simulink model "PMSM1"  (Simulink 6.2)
settings: Solver=ode45  StartTime=0  StopTime=0.2  FixedStep=0.000001  RelTol=1e-3
undefined symbols (not defined in the file or in its folder): di, DiscIntNeverNeededParam, Element, J, Lsx, Lsy, p, Psim, Rs, Symmetrized, Ts, Udc, Warning
libraries: simulink x4

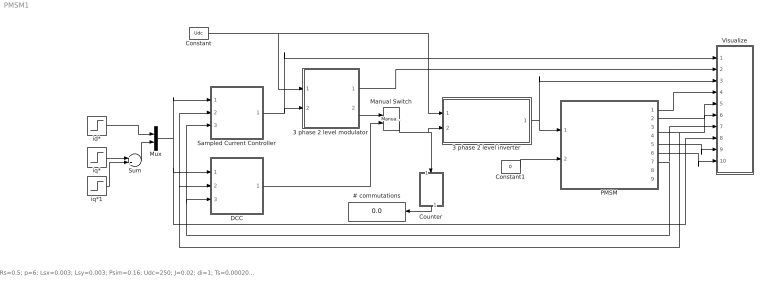
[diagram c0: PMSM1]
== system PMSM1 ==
  note: Rs=0.5; p=6; Lsx=0.003; Lsy=0.003; Psim=0.16; Udc=250; J=0.02; di=1; Ts=0.0002083;
  # commutations : Display
  3 phase 2 level inverter : Subsystem
  3 phase 2 level modulator : Subsystem  mask{type=Symmetrized, Random=Fixed frequency, Ts=Ts}
      mask prompts: type "Sinus, Symmetrized or Minimum switch modulation"; Random "Fixed or random modulation?"; Ts "Sampling interval"
      mask help: Carrier Wave modulator that uses either fixed frequency modulation or random modulation. The fixed frequency modulation uses 1/(2Ts) as modulation frequency. The random modulation selects the modulatio frequency by random every sampling instant. The selection uses either 1/Ts, 1/(2Ts) or 1/(3Ts) as carrier wave frequency.
  Constant : Constant  Value=Udc
  Constant1 : Constant  Value=0
  Counter : Subsystem  Orientation=down
  DCC : Subsystem
  Manual Switch : simulink/Signal Routing/Manual Switch  sw=1  action=0
  Mux : Mux  Inputs=2
  PMSM : Subsystem  mask{Psim=Psim, p=p, Rs=Rs, isy=[0 1], psisy=[0 Lsy], isx=[0 1], psisx=[0 Lsx], J=J}
      mask prompts: p "Number of poles"; Rs "Stator resistance"; isy "y-axis current vector"; psisy "y-axis flux vector"; isx "x-axis current vector"; psisx "x-axis flux vector"; J "Inertia"
  Sampled Current Controller : Subsystem  mask{R=Rs, Lx=Lsx, Ly=Lsy, Kp=[(Lsx/Ts+Rs/2) (Lsy/Ts+Rs/2)]', Ti=[(Lsx/Rs+Ts/2) (Lsy/Rs+Ts/2)]', Ts=Ts, Umax=Udc, Umin=-Udc, SlowFast=Fast computer}
      mask prompts: R "Load resistance"; Lx "x-axis load inductance"; Ly "y-axis load inductance"; Kp "Controller gain"; Ti "Integral Time Constant"; Ts "Sampling time [s]"; Umax "Max output signal"; Umin "Min output signal"; SlowFast "Controller type"
  Sum : Sum
  Visualize : Subsystem
  id* : Step  Time=0.0105  After=0  SampleTime=0
  iq* : Step  Time=0.0055  After=10  SampleTime=0
  iq*1 : Step  Time=0.05  After=-5  SampleTime=0
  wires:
  3 phase 2 level inverter/1(va,b,c) -> Visualize/3(v), PMSM/1(vabc)
  Sampled Current Controller/1(u*) -> 3 phase 2 level modulator/2(uabc*), Visualize/1(u*)
  Constant/1 -> 3 phase 2 level inverter/1(Udc), 3 phase 2 level modulator/1(Udc)
  Counter/1(#) -> # commutations/1
  3 phase 2 level modulator/2(sa,b,c) -> Manual Switch/1
  Manual Switch/1 -> 3 phase 2 level inverter/2(sa,b,c), Counter/1(sa,b,c)
  DCC/1(sa,b,c) -> Manual Switch/2
  3 phase 2 level modulator/1(mod) -> Visualize/2(mod)
  id*/1 -> Mux/1
  Mux/1 -> Sampled Current Controller/1(Ref_dq), DCC/1(Ref_dq), Visualize/8(i*dq)
  PMSM/7(theta_el) -> Visualize/7(theta), Sampled Current Controller/3(thetaR), DCC/3(thetaR)
  Constant1/1 -> PMSM/2(Tl)
  PMSM/1(uabc) -> Visualize/4("u ")
  PMSM/4(is) -> Visualize/6(i), DCC/2(Act_ab), Sampled Current Controller/2(Act_ab)
  PMSM/2(exy) -> Visualize/5(e)
  PMSM/5(T_mech) -> Visualize/9(Tmech)
  PMSM/6(w_mech) -> Visualize/10(wmech)
  iq*/1 -> Sum/1
  iq*1/1 -> Sum/2
  Sum/1 -> Mux/2

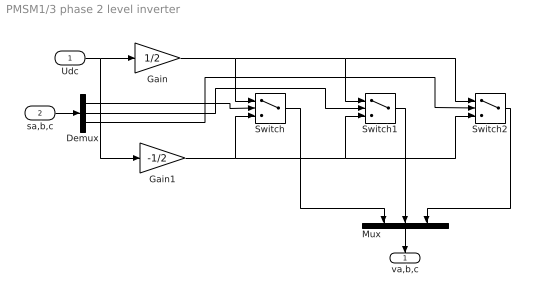
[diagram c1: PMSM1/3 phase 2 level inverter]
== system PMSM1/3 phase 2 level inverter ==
  Udc : Inport  Port=1  LatchInput=off
  sa,b,c : Inport  Port=2  LatchInput=off
  Demux : Demux  Outputs=3
  Gain : Gain  Gain=1/2
  Gain1 : Gain  Gain=-1/2
  Mux : Mux  Orientation=down  Inputs=3
  Switch : Switch
  Switch1 : Switch
  Switch2 : Switch
  va,b,c : Outport  Orientation=down  InitialOutput=0
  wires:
  Gain/1 -> Switch/1, Switch1/1, Switch2/1
  Gain1/1 -> Switch/3, Switch1/3, Switch2/3
  Udc/1 -> Gain1/1, Gain/1
  sa,b,c/1 -> Demux/1
  Demux/1 -> Switch/2
  Demux/2 -> Switch1/2
  Demux/3 -> Switch2/2
  Switch/1 -> Mux/1
  Switch1/1 -> Mux/2
  Switch2/1 -> Mux/3
  Mux/1 -> va,b,c/1

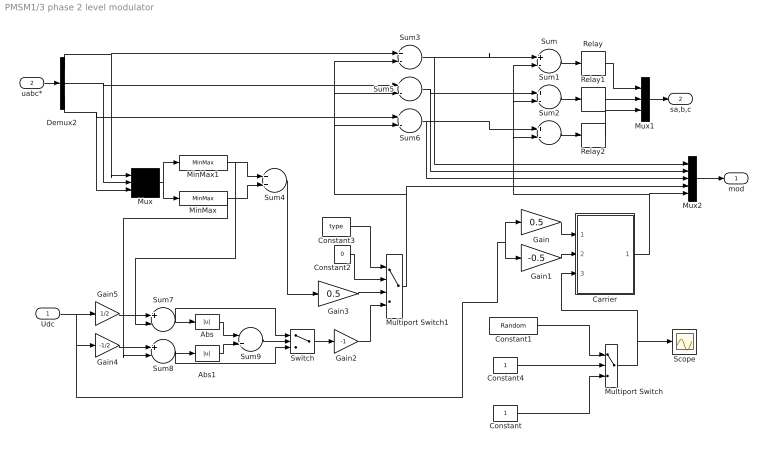
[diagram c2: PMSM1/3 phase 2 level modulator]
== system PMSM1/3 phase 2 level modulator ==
  Udc : Inport  Port=1  LatchInput=off
  uabc* : Inport  Port=2  LatchInput=off
  Abs : Abs
  Abs1 : Abs
  Carrier : Subsystem
  Constant : Constant
  Constant1 : Constant  Value=Random
  Constant2 : Constant  Value=0
  Constant3 : Constant  Value=type
  Constant4 : Constant
  Demux2 : Demux  Outputs=3
  Gain : Gain  Gain=0.5
  Gain1 : Gain  Gain=-0.5
  Gain2 : Gain  Gain=-1
  Gain3 : Gain  Gain=0.5
  Gain4 : Gain  Gain=-1/2
  Gain5 : Gain  Gain=1/2
  MinMax : MinMax
  MinMax1 : MinMax  Function=max
  Multiport Switch : MultiPortSwitch  Inputs=2
  Multiport Switch1 : MultiPortSwitch  Inputs=3
  Mux : Mux  Inputs=3
  Mux1 : Mux  Inputs=3
  Mux2 : Mux  Inputs=5
  Relay : Relay  OffOutputValue=-1
  Relay1 : Relay  OffOutputValue=-1
  Relay2 : Relay  OffOutputValue=-1
  Scope : Scope
  Sum{,1..3,5..8} (8 alike) : Sum  Inputs=+-
  Sum4 : Sum
  Sum9 : Sum  Inputs=-+
  Switch : Switch
  mod : Outport  InitialOutput=0
  sa,b,c : Outport  Port=2  InitialOutput=0
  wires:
  Carrier/1(um) -> Sum2/2, Sum1/2, Sum/2, Mux2/5
  Gain1/1 -> Carrier/2(Umin)
  Gain/1 -> Carrier/1(Umax)
  Sum/1 -> Relay/1
  Relay1/1 -> Mux1/2
  Sum1/1 -> Relay1/1
  Relay2/1 -> Mux1/3
  Sum2/1 -> Relay2/1
  Constant/1 -> Multiport Switch/3
  Multiport Switch/1 -> Carrier/3(x), Scope/1
  Constant1/1 -> Multiport Switch/1
  Sum3/1 -> Mux2/1, Sum/1
  Sum5/1 -> Mux2/2, Sum1/1
  Sum6/1 -> Mux2/3, Sum2/1
  Demux2/1 -> Sum3/1, Mux/1
  Demux2/2 -> Sum5/1, Mux/2
  Demux2/3 -> Sum6/1, Mux/3
  Mux/1 -> MinMax1/1, MinMax/1
  MinMax1/1 -> Sum4/1, Sum7/2
  MinMax/1 -> Sum4/2, Sum8/2
  Udc/1 -> Gain5/1, Gain4/1, Gain1/1, Gain/1
  Gain4/1 -> Sum8/1
  Sum7/1 -> Abs/1, Switch/1
  Sum8/1 -> Abs1/1, Switch/3
  Abs/1 -> Sum9/1
  Abs1/1 -> Sum9/2
  Sum9/1 -> Switch/2
  Sum4/1 -> Gain3/1
  Switch/1 -> Gain2/1
  Constant3/1 -> Multiport Switch1/1
  Constant2/1 -> Multiport Switch1/2
  Gain3/1 -> Multiport Switch1/3
  Gain2/1 -> Multiport Switch1/4
  Multiport Switch1/1 -> Sum5/2, Sum3/2, Sum6/2, Mux2/4
  Gain5/1 -> Sum7/1
  uabc*/1 -> Demux2/1
  Relay/1 -> Mux1/1
  Mux1/1 -> sa,b,c/1
  Mux2/1 -> mod/1
  Constant4/1 -> Multiport Switch/2

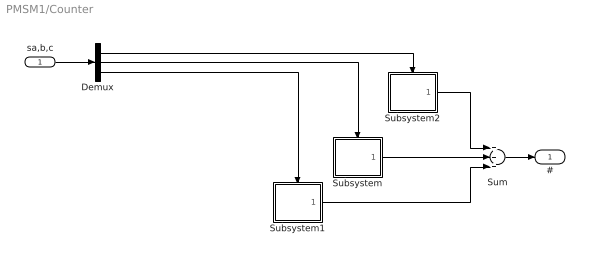
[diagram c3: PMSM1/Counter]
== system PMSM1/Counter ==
  sa,b,c : Inport  Port=1  LatchInput=off
  Demux : Demux  Outputs=3
  Subsystem : Subsystem  TreatAsAtomicUnit=on
  Subsystem1 : Subsystem  TreatAsAtomicUnit=on
  Subsystem2 : Subsystem  TreatAsAtomicUnit=on
  Sum : Sum  Inputs=+++
  # : Outport
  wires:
  Sum/1 -> #/1
  Subsystem/1(Out1) -> Sum/2
  Subsystem2/1(Out1) -> Sum/1
  Subsystem1/1(Out1) -> Sum/3
  sa,b,c/1 -> Demux/1
  Demux/2 -> Subsystem/Trigger
  Demux/3 -> Subsystem1/Trigger
  Demux/1 -> Subsystem2/Trigger

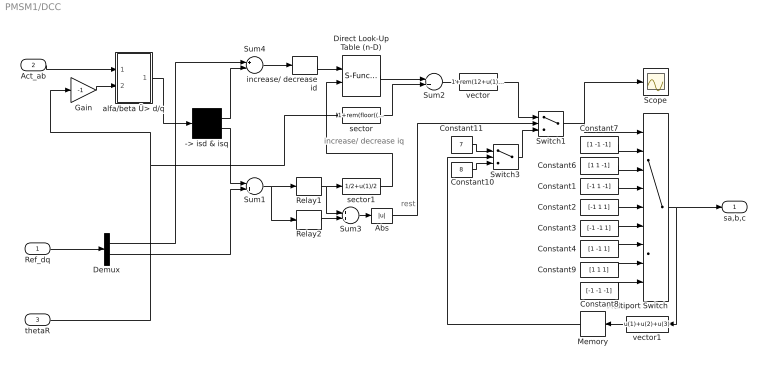
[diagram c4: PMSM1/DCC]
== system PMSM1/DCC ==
  note: increase/ decrease iq
  note: rest
  Ref_dq : Inport  Port=1  LatchInput=off
  Act_ab : Inport  Port=2  LatchInput=off
  thetaR : Inport  Port=3  LatchInput=off
  -> isd & isq : Demux  Outputs=2
  Abs : Abs
  Constant1 : Constant  Value=[-1 1 -1]
  Constant10 : Constant  Value=8
  Constant11 : Constant  Value=7
  Constant2 : Constant  Value=[-1 1 1]
  Constant3 : Constant  Value=[-1 -1 1]
  Constant4 : Constant  Value=[1 -1 1]
  Constant6 : Constant  Value=[1 1 -1]
  Constant7 : Constant  Value=[1 -1 -1]
  Constant8 : Constant  Value=[-1 -1 -1]
  Constant9 : Constant  Value=[1 1 1]
  Demux : Demux  Outputs=2
  Direct Look-Up Table (n-D) : S-Function  FunctionName=sfun_nddirectlook  Parameters=numInputs,mxTable,clipFlag,tabIsInput,numTDims  mask(LookupNDDirect){maskTabDims=2, explicitNumDims=1, outDims=Element, tabIsInput=off, mxTable=[4 2;5 1], clipFlag=Warning}
      mask prompts: maskTabDims "Number of table dimensions:"; explicitNumDims "Explicit number of table dimensions:"; outDims "Inputs select this object from table:"; tabIsInput "Make table an input"; mxTable "Table data:"; clipFlag "Action for out of range input:"
      mask help: Table member selection. Inputs are zero-based indices into the table, e.g., an input of 3 returns the fourth element in that dimension. Block can also be used to select a column or 2-D matrix out of the table.
      mask init:
      | if tabIsInput == 1
      |   tWhat = ' T';
      |   yT = 1/(3+maskTabDims-outDims);
      | else
      |   tWhat = ' ';
      |   yT = 0;
      | end
      | if maskTabDims >= 5
      |   numTDims = explicitNumDims;
      | else
      |   numTDims = maskTabDims;
      | end
      | numInputs =  numTDims - (outDims-1);
      | if strcmp(get_param(bdroot(gcb),'BlockDiagramType'),'library')
      |   dimsChar = 'n';
      | else
      |   dimsChar = sprintf('%d',numTDims);
      | end
      | [x,y] = nddirectico('plotdata', numTDims, tabIsInput, outDims);
      | xp = x((end-3):end); yp = y((end-3):end);
      | x = x(1:(end-4)); y = y(1:(end-4));
  Gain : Gain  Gain=-1
  Memory : Memory  Orientation=left
  Multiport Switch : MultiPortSwitch  Inputs=8
  Relay1 : Relay  OnSwitchValue=di/2  OffSwitchValue=-di/2  OffOutputValue=-1
  Relay2 : Relay  OnSwitchValue=1.3*di/2  OffSwitchValue=-1.3*di/2  OffOutputValue=-1
  Scope : Scope
  Sum1 : Sum  Inputs=-+
  Sum2 : Sum
  Sum3 : Sum
  Sum4 : Sum  Inputs=+-
  Switch1 : Switch  Threshold=1
  Switch3 : Switch  Threshold=1
  alfa/beta Ü> d/q : Subsystem
  increase/ decrease id : Relay  OnSwitchValue=di/2  OffSwitchValue=-di/2
  sector : Fcn  Expr=1+rem(floor((2*pi+u(1)+pi/6)/(pi/3+eps)),6)
  sector1 : Fcn  Expr=1/2+u(1)/2
  vector : Fcn  Expr=1+rem(12+u(1)-1,6)
  vector1 : Fcn  Orientation=left  Expr=u(1)+u(2)+u(3)
  sa,b,c : Outport
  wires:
  Gain/1 -> alfa/beta Ü> d/q/2(angle)
  Act_ab/1 -> alfa/beta Ü> d/q/1(vect)
  alfa/beta Ü> d/q/1(Out) -> -> isd & isq/1
  -> isd & isq/1 -> Sum4/2
  Multiport Switch/1 -> vector1/1, sa,b,c/1
  Switch1/1 -> Multiport Switch/1, Scope/1
  vector/1 -> Switch1/1
  Sum4/1 -> increase/ decrease id/1
  Sum2/1 -> vector/1
  vector1/1 -> Memory/1
  -> isd & isq/2 -> Sum1/1
  Constant10/1 -> Switch3/3
  Constant11/1 -> Switch3/1
  Memory/1 -> Switch3/2
  Switch3/1 -> Switch1/3
  Relay1/1 -> Sum3/1, sector1/1
  Relay2/1 -> Sum3/2
  Sum3/1 -> Abs/1
  Sum1/1 -> Relay1/1, Relay2/1
  Abs/1 -> Switch1/2
  increase/ decrease id/1 -> Direct Look-Up Table (n-D)/1
  sector1/1 -> Direct Look-Up Table (n-D)/2
  sector/1 -> Sum2/2
  Direct Look-Up Table (n-D)/1 -> Sum2/1
  Constant6/1 -> Multiport Switch/3
  Constant7/1 -> Multiport Switch/2
  Constant8/1 -> Multiport Switch/9
  Constant9/1 -> Multiport Switch/8
  Constant1/1 -> Multiport Switch/4
  Constant2/1 -> Multiport Switch/5
  Constant3/1 -> Multiport Switch/6
  Constant4/1 -> Multiport Switch/7
  Ref_dq/1 -> Demux/1
  Demux/1 -> Sum4/1
  Demux/2 -> Sum1/2
  thetaR/1 -> Gain/1, sector/1

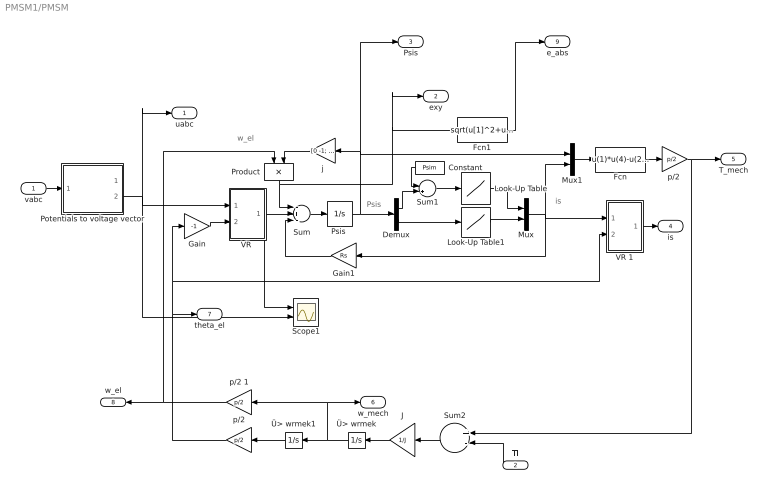
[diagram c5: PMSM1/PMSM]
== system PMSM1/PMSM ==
  note: w_el
  note: Psis
  note: is
  vabc : Inport  Port=1  LatchInput=off
  Tl : Inport  Orientation=left  Port=2  LatchInput=off
  Constant : Constant  Orientation=left  Value=Psim
  Demux : Demux  Outputs=2
  Fcn : Fcn  Expr=u(1)*u(4)-u(2)*u(3)
  Fcn1 : Fcn  Expr=sqrt(u[1]^2+u[2]^2)
  Gain : Gain  Gain=-1
  Gain1 : Gain  Orientation=left  Gain=Rs
  J : Gain  Orientation=left  Gain=1/J
  Look-Up Table : Lookup  InputValues=psisx  OutputValues=isx
  Look-Up Table1 : Lookup  InputValues=psisy  OutputValues=isy
  Mux : Mux  Inputs=2
  Mux1 : Mux  Inputs=2
  Potentials to voltage vector : Subsystem
  Product : Product  Orientation=down
  "Psis " : Integrator  InitialCondition=[Psim 0]'  LimitOutput=on  UpperSaturationLimit=[2*Psim Psim*2]'  LowerSaturationLimit=[Psim/20 0]'
  Scope1 : Scope  NumInputPorts=2
  Sum : Sum  Inputs=-+-
  Sum1 : Sum  Inputs=-+
  Sum2 : Sum  Orientation=left  Inputs=+-
  "VR " : Subsystem
  VR 1 : Subsystem
  j : Gain  Orientation=left  Gain=[0 -1; 1 0]  Multiplication=Matrix(K*u)
  p/2 : Gain  Orientation=left  Gain=p/2  Multiplication=Matrix(K*u)
  "p/2 " : Gain  Gain=p/2  Multiplication=Matrix(K*u)
  p/2 1 : Gain  Orientation=left  Gain=p/2  Multiplication=Matrix(K*u)
  Ü> wrmek : Integrator  Orientation=left
  Ü> wrmek1 : Integrator  Orientation=left
  uabc : Outport
  exy : Outport  Port=2
  Psis : Outport  Port=3
  is : Outport  Port=4
  T_mech : Outport  Port=5
  w_mech : Outport  Port=6
  theta_el : Outport  Port=7
  w_el : Outport  Orientation=left  Port=8
  e_abs : Outport  Port=9
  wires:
  VR 1/1(Out) -> is/1
  Ü> wrmek/1 -> Ü> wrmek1/1, p/2 1/1, w_mech/1
  Fcn1/1 -> e_abs/1
  p/2 1/1 -> w_el/1, Product/1
  Tl/1 -> Sum2/2
  Ü> wrmek1/1 -> p/2/1
  Sum2/1 -> J/1
  J/1 -> Ü> wrmek/1
  vabc/1 -> Potentials to voltage vector/1(In1)
  Potentials to voltage vector/2(uab) -> "VR "/1(vect), uabc/1, Scope1/2
  "p/2 "/1 -> Sum2/1, T_mech/1
  Gain/1 -> "VR "/2(angle)
  Sum/1 -> "Psis "/1
  "Psis "/1 -> Demux/1, j/1, Mux1/1, Psis/1
  Demux/1 -> Sum1/2
  Demux/2 -> Look-Up Table1/1
  Look-Up Table/1 -> Mux/1
  Look-Up Table1/1 -> Mux/2
  Mux/1 -> Mux1/2, Gain1/1, VR 1/1(vect)
  Mux1/1 -> Fcn/1
  Constant/1 -> Sum1/1
  Sum1/1 -> Look-Up Table/1
  Gain1/1 -> Sum/3
  "VR "/1(Out) -> Sum/2, Scope1/1
  Product/1 -> Sum/1, Fcn1/1, exy/1
  Fcn/1 -> "p/2 "/1
  j/1 -> Product/2
  p/2/1 -> theta_el/1, Gain/1, VR 1/2(angle)

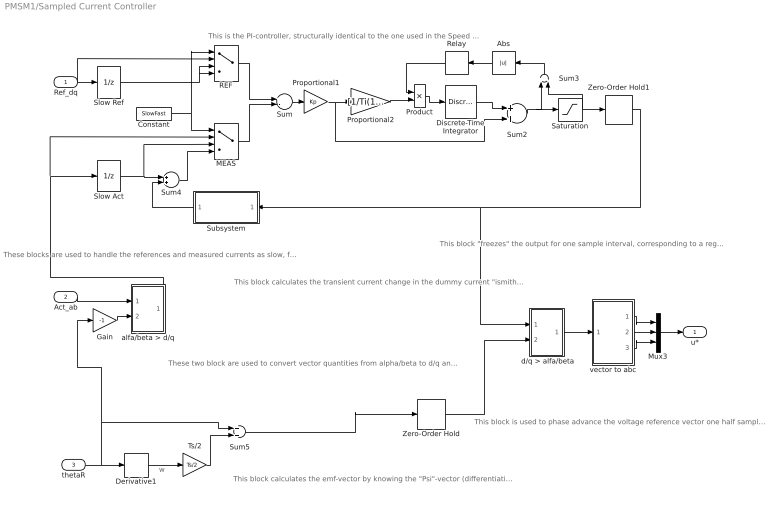
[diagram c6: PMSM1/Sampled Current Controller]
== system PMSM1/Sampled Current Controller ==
  note: These blocks are used to handle the references and measured currents as slow, fast or fast computer with Smith predictor.
  note: This block calculates the transient current change in the dummy current "ismith" The smith predictor calculates the current change that would have been measured if the computer was "fast", i.e. without the delay that a slow computer has. The calculated current change equals the real current change, but informing the controller one sampling interval earlier, thus allowing a high (deadbeat) gain.
  note: This is the PI-controller, structurally identical to the one used in the Speed Controller
  note: This block "freezes" the output for one sample interval, corresponding to a register in a microcontroller where the reference voltages are written once every sampling inteval.
  note: These two block are used to convert vector quantities from alpha/beta to d/q and back again. Note that they are identical, but use the angle with opposite sign.
  note: This block calculates the emf-vector by knowing the "Psi"-vector (differentiation) and calculates the emf- components in the d/q-plane (ideally there is only "eq" whilse "ed"=0). It alse calculates the angle of the "Psi"- vector, used to orient the d/q-plane.
  note: This block is used to phase advance the voltage reference vector one half sample period. It is done to compensate for the fact that the "reality" is turning during the same sample period as the voltage references are being held constant. In the beginning of the sample period, the voltage reference will be 1/2 sample period ahead of reality, and in the end of the sample period it will be 1/2 period behind. In average, it will be in the correct position relative to reality.
  note: w
  Ref_dq : Inport  Port=1  LatchInput=off
  Act_ab : Inport  Port=2  LatchInput=off
  thetaR : Inport  Port=3  LatchInput=off
  " d/q > alfa/beta" : Subsystem
  Abs : Abs  Orientation=left
  Constant : Constant  Value=SlowFast
  Derivative1 : Derivative
  Discrete-Time Integrator : DiscreteIntegrator  SampleTime=Ts  LimitOutput=on  UpperSaturationLimit=Umax  LowerSaturationLimit=Umin  ICPrevOutput=DiscIntNeverNeededParam  ICPrevScaledInput=DiscIntNeverNeededParam
  Gain : Gain  Gain=-1
  MEAS : MultiPortSwitch  Inputs=3
  Mux3 : Mux  Inputs=3
  Product : Product
  Proportional1 : Gain  Gain=Kp
  Proportional2 : Gain  Gain=[1/Ti(1) 1/Ti(2)]
  REF : MultiPortSwitch  Inputs=3
  Relay : Relay  Orientation=left  OnOutputValue=0  OffOutputValue=1
  Saturation : Saturate  UpperLimit=Umax  LowerLimit=Umin
  Slow Act : UnitDelay  SampleTime=Ts
  Slow Ref : UnitDelay  SampleTime=Ts
  Subsystem : Subsystem  Orientation=left
  Sum : Sum  Inputs=+-
  Sum2 : Sum
  Sum3 : Sum  Orientation=up  Inputs=+-
  Sum4 : Sum
  Sum5 : Sum
  Ts/2 : Gain  Gain=Ts/2  Multiplication=Matrix(K*u)
  Zero-Order Hold : ZeroOrderHold  SampleTime=Ts
  Zero-Order Hold1 : ZeroOrderHold  SampleTime=Ts
  alfa/beta > d/q : Subsystem
  vector to abc : Subsystem
  u* : Outport
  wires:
  Discrete-Time Integrator/1 -> Sum2/1
  Proportional1/1 -> Proportional2/1, Sum2/2
  Sum/1 -> Proportional1/1
  Sum2/1 -> Saturation/1, Sum3/1
  Saturation/1 -> Zero-Order Hold1/1, Sum3/2
  Proportional2/1 -> Product/2
  Product/1 -> Discrete-Time Integrator/1
  Relay/1 -> Product/1
  Ref_dq/1 -> REF/2, Slow Ref/1
  Zero-Order Hold1/1 -> Subsystem/1(u), " d/q > alfa/beta"/1(vect)
  Slow Act/1 -> Sum4/1, MEAS/3
  Subsystem/1(di_smith) -> Sum4/2
  Constant/1 -> MEAS/1, REF/1
  Slow Ref/1 -> REF/3, REF/4
  REF/1 -> Sum/1
  Sum4/1 -> MEAS/4
  MEAS/1 -> Sum/2
  Sum3/1 -> Abs/1
  Abs/1 -> Relay/1
  Gain/1 -> alfa/beta > d/q/2(angle)
  Act_ab/1 -> alfa/beta > d/q/1(vect)
  Sum5/1 -> Zero-Order Hold/1
  Zero-Order Hold/1 -> " d/q > alfa/beta"/2(angle)
  " d/q > alfa/beta"/1(Out) -> vector to abc/1(vect)
  vector to abc/1(a) -> Mux3/1
  vector to abc/2(b) -> Mux3/2
  vector to abc/3(c) -> Mux3/3
  alfa/beta > d/q/1(Out) -> Slow Act/1, MEAS/2
  Mux3/1 -> u*/1
  thetaR/1 -> Derivative1/1, Gain/1, Sum5/1
  Derivative1/1 -> Ts/2/1
  Ts/2/1 -> Sum5/2

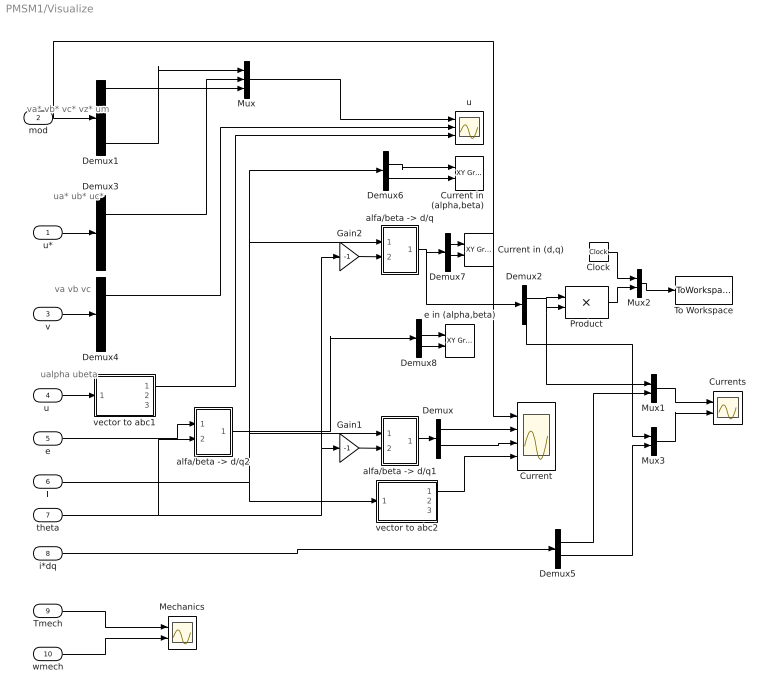
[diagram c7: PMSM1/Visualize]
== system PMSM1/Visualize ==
  note: va* vb* vc* vz* um
  note: ua* ub* uc*
  note: ualpha ubeta
  note: va vb vc
  u* : Inport  Port=1  LatchInput=off
  mod : Inport  Port=2  LatchInput=off
  v : Inport  Port=3  LatchInput=off
  "u " : Inport  Port=4  LatchInput=off
  e : Inport  Port=5  LatchInput=off
  i : Inport  Port=6  LatchInput=off
  theta : Inport  Port=7  LatchInput=off
  i*dq : Inport  Port=8  LatchInput=off
  Tmech : Inport  Port=9  LatchInput=off
  wmech : Inport  Port=10  LatchInput=off
  Clock : Clock
  Current : Scope  NumInputPorts=4
  Current in (alpha,beta) : simulink/Sinks/XY Graph  xmin=-20  xmax=20  ymin=-20  ymax=20  st=-1
  Current in (d,q) : simulink/Sinks/XY Graph  xmin=-20  xmax=20  ymin=-20  ymax=20  st=-1
  Currents : Scope  NumInputPorts=2
  Demux{,2,5..8} (6 alike) : Demux  Outputs=2
  Demux1 : Demux  Outputs=5
  Demux3 : Demux  Outputs=3
  Demux4 : Demux  Outputs=3
  Gain1 : Gain  Gain=-1
  Gain2 : Gain  Gain=-1
  Mechanics : Scope  NumInputPorts=2
  Mux : Mux  Inputs=3
  Mux1 : Mux  Inputs=2
  Mux2 : Mux  Inputs=2
  Mux3 : Mux  Inputs=2
  Product : Product
  To Workspace : ToWorkspace  VariableName=f1  SampleTime=-1  SaveFormat=Array
  "alfa/beta -> d/q" : Subsystem
  "alfa/beta -> d/q1" : Subsystem
  "alfa/beta -> d/q2" : Subsystem
  e in (alpha,beta) : simulink/Sinks/XY Graph  xmin=-300  xmax=300  ymin=-300  ymax=300  st=-1
  u : Scope  NumInputPorts=3
  vector to abc1 : Subsystem
  vector to abc2 : Subsystem
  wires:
  Gain2/1 -> "alfa/beta -> d/q"/2(angle)
  Gain1/1 -> "alfa/beta -> d/q1"/2(angle)
  "alfa/beta -> d/q1"/1(Out) -> Demux/1
  Demux/1 -> Current/2
  Demux/2 -> Current/3
  vector to abc2/1(a) -> Current/4
  mod/1 -> Demux1/1, Current/1
  "alfa/beta -> d/q"/1(Out) -> Demux2/1, Demux7/1
  Demux1/5 -> Mux/1
  Demux1/1 -> Mux/3
  Mux/1 -> u/1
  u*/1 -> Demux3/1
  "u "/1 -> vector to abc1/1(vect)
  Demux3/1 -> Mux/2
  v/1 -> Demux4/1
  Demux4/1 -> u/2
  vector to abc1/1(a) -> u/3
  i/1 -> "alfa/beta -> d/q"/1(vect), Demux6/1, "alfa/beta -> d/q1"/1(vect), vector to abc2/1(vect)
  theta/1 -> Gain1/1, Gain2/1, "alfa/beta -> d/q2"/2(angle)
  Clock/1 -> Mux2/1
  Product/1 -> Mux2/2
  Mux2/1 -> To Workspace/1
  Demux2/1 -> Product/1, Product/2, Mux1/1
  i*dq/1 -> Demux5/1
  Demux5/1 -> Mux1/2
  Demux2/2 -> Mux3/1
  Demux5/2 -> Mux3/2
  Mux3/1 -> Currents/2
  Mux1/1 -> Currents/1
  e/1 -> "alfa/beta -> d/q2"/1(vect)
  "alfa/beta -> d/q2"/1(Out) -> Demux8/1
  Tmech/1 -> Mechanics/1
  wmech/1 -> Mechanics/2
  Demux6/1 -> Current in (alpha,beta)/1
  Demux6/2 -> Current in (alpha,beta)/2
  Demux7/1 -> Current in (d,q)/1
  Demux7/2 -> Current in (d,q)/2
  Demux8/1 -> e in (alpha,beta)/1
  Demux8/2 -> e in (alpha,beta)/2

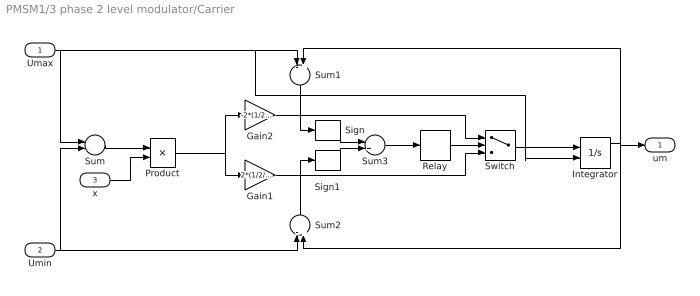
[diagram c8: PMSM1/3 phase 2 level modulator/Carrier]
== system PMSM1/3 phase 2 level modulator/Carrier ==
  Umax : Inport  Port=1  LatchInput=off
  Umin : Inport  Port=2  LatchInput=off
  x : Inport  Port=3  LatchInput=off
  Gain1 : Gain  Gain=2*(1/2/Ts)
  Gain2 : Gain  Gain=-2*(1/2/Ts)
  Integrator : Integrator  InitialConditionSource=external
  Product : Product
  Relay : Relay  OnSwitchValue=1  OffSwitchValue=-1  OffOutputValue=-1
  Sign : Signum
  Sign1 : Signum
  Sum : Sum  Inputs=+-
  Sum1 : Sum  Orientation=down  Inputs=-+
  Sum2 : Sum  Orientation=up  Inputs=-+
  Sum3 : Sum
  Switch : Switch
  um : Outport
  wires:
  Switch/1 -> Integrator/1
  Umax/1 -> Sum/1, Sum1/1, Integrator/2
  Umin/1 -> Sum/2, Sum2/1
  Gain2/1 -> Switch/1
  Gain1/1 -> Switch/3
  Integrator/1 -> Sum1/2, um/1, Sum2/2
  Sum1/1 -> Sign/1
  Sum2/1 -> Sign1/1
  Sign/1 -> Sum3/1
  Sign1/1 -> Sum3/2
  Sum3/1 -> Relay/1
  Relay/1 -> Switch/2
  Sum/1 -> Product/1
  Product/1 -> Gain2/1, Gain1/1
  x/1 -> Product/2

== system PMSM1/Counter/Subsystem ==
  Trigger : TriggerPort  TriggerType=either
  Constant : Constant
  Memory : Memory  Orientation=left  InheritSampleTime=on
  Sum : Sum
  Out1 : Outport
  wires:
  Sum/1 -> Memory/1, Out1/1
  Memory/1 -> Sum/2
  Constant/1 -> Sum/1

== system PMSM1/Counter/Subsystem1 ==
  Trigger : TriggerPort  TriggerType=either
  Constant : Constant
  Memory : Memory  Orientation=left  InheritSampleTime=on
  Sum : Sum
  Out1 : Outport
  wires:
  Constant/1 -> Sum/1
  Memory/1 -> Sum/2
  Sum/1 -> Memory/1, Out1/1

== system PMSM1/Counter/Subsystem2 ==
  Trigger : TriggerPort  TriggerType=either
  Constant : Constant
  Memory : Memory  Orientation=left  InheritSampleTime=on
  Sum : Sum
  Out1 : Outport
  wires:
  Sum/1 -> Memory/1, Out1/1
  Memory/1 -> Sum/2
  Constant/1 -> Sum/1

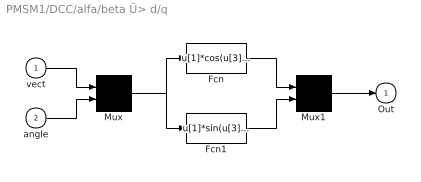
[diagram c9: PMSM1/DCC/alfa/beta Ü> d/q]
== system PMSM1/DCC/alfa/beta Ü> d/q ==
  vect : Inport  Port=1  LatchInput=off
  angle : Inport  Port=2  LatchInput=off
  Fcn : Fcn  Expr=u[1]*cos(u[3])-u[2]*sin(u[3])
  Fcn1 : Fcn  Expr=u[1]*sin(u[3])+u[2]*cos(u[3])
  Mux : Mux  Inputs=2
  Mux1 : Mux  Inputs=2
  Out : Outport  InitialOutput=0
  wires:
  vect/1 -> Mux/1
  angle/1 -> Mux/2
  Mux/1 -> Fcn/1, Fcn1/1
  Fcn/1 -> Mux1/1
  Fcn1/1 -> Mux1/2
  Mux1/1 -> Out/1

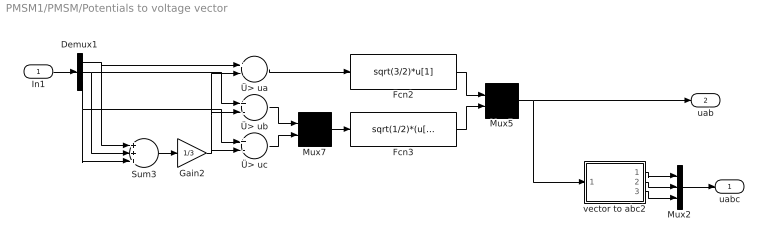
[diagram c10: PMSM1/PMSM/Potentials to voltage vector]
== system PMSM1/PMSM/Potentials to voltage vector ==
  In1 : Inport  Port=1  LatchInput=off
  Demux1 : Demux  Outputs=3
  Fcn2 : Fcn  Expr=sqrt(3/2)*u[1]
  Fcn3 : Fcn  Expr=sqrt(1/2)*(u[1]-u[2])
  Gain2 : Gain  Gain=1/3
  Mux2 : Mux  Inputs=3
  Mux5 : Mux  Inputs=2
  Mux7 : Mux  Inputs=2
  Sum3 : Sum  Inputs=+++
  vector to abc2 : Subsystem
  Ü> ua : Sum  Inputs=+-
  Ü> ub : Sum  Inputs=+-
  Ü> uc : Sum  Inputs=+-
  uabc : Outport
  uab : Outport  Port=2
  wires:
  Fcn3/1 -> Mux5/2
  Fcn2/1 -> Mux5/1
  Mux7/1 -> Fcn3/1
  Ü> uc/1 -> Mux7/2
  Ü> ub/1 -> Mux7/1
  Ü> ua/1 -> Fcn2/1
  Gain2/1 -> Ü> uc/2, Ü> ub/2, Ü> ua/2
  Demux1/2 -> Ü> ub/1, Sum3/2
  Sum3/1 -> Gain2/1
  Demux1/3 -> Ü> uc/1, Sum3/3
  Demux1/1 -> Ü> ua/1, Sum3/1
  In1/1 -> Demux1/1
  Mux5/1 -> uab/1, vector to abc2/1(vect)
  vector to abc2/1(a) -> Mux2/1
  vector to abc2/2(b) -> Mux2/2
  vector to abc2/3(c) -> Mux2/3
  Mux2/1 -> uabc/1

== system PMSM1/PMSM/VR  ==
  vect : Inport  Port=1  LatchInput=off
  angle : Inport  Port=2  LatchInput=off
  Fcn : Fcn  Expr=u[1]*cos(u[3])-u[2]*sin(u[3])
  Fcn1 : Fcn  Expr=u[1]*sin(u[3])+u[2]*cos(u[3])
  Mux : Mux  Inputs=2
  Mux1 : Mux  Inputs=2
  Out : Outport  InitialOutput=0
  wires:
  Mux1/1 -> Out/1
  Fcn1/1 -> Mux1/2
  Fcn/1 -> Mux1/1
  Mux/1 -> Fcn1/1, Fcn/1
  angle/1 -> Mux/2
  vect/1 -> Mux/1

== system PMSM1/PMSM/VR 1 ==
  vect : Inport  Port=1  LatchInput=off
  angle : Inport  Port=2  LatchInput=off
  Fcn : Fcn  Expr=u[1]*cos(u[3])-u[2]*sin(u[3])
  Fcn1 : Fcn  Expr=u[1]*sin(u[3])+u[2]*cos(u[3])
  Mux : Mux  Inputs=2
  Mux1 : Mux  Inputs=2
  Out : Outport  InitialOutput=0
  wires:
  vect/1 -> Mux/1
  angle/1 -> Mux/2
  Mux/1 -> Fcn/1, Fcn1/1
  Fcn/1 -> Mux1/1
  Fcn1/1 -> Mux1/2
  Mux1/1 -> Out/1

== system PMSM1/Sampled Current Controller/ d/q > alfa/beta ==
  vect : Inport  Port=1  LatchInput=off
  angle : Inport  Port=2  LatchInput=off
  Fcn : Fcn  Expr=u[1]*cos(u[3])-u[2]*sin(u[3])
  Fcn1 : Fcn  Expr=u[1]*sin(u[3])+u[2]*cos(u[3])
  Mux : Mux  Inputs=2
  Mux1 : Mux  Inputs=2
  Out : Outport  InitialOutput=0
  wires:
  Mux1/1 -> Out/1
  Fcn1/1 -> Mux1/2
  Fcn/1 -> Mux1/1
  Mux/1 -> Fcn1/1, Fcn/1
  angle/1 -> Mux/2
  vect/1 -> Mux/1

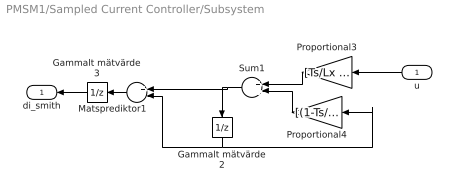
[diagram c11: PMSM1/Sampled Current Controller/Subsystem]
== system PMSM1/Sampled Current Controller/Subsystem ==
  u : Inport  Orientation=left  Port=1  LatchInput=off
  Gammalt mätvärde2 : UnitDelay  Orientation=down  SampleTime=Ts
  Gammalt mätvärde3 : UnitDelay  Orientation=left  SampleTime=Ts
  Matsprediktor1 : Sum  Orientation=left  Inputs=+-
  Proportional3 : Gain  Orientation=left  Gain=[Ts/Lx Ts/Ly]
  Proportional4 : Gain  Orientation=left  Gain=[(1-Ts/(Lx/R)) (1-Ts/(Ly/R))]
  Sum1 : Sum  Orientation=left
  di_smith : Outport  Orientation=left
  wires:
  Proportional3/1 -> Sum1/1
  Proportional4/1 -> Sum1/2
  Sum1/1 -> Gammalt mätvärde2/1, Matsprediktor1/1
  u/1 -> Proportional3/1
  Matsprediktor1/1 -> Gammalt mätvärde3/1
  Gammalt mätvärde3/1 -> di_smith/1
  Gammalt mätvärde2/1 -> Proportional4/1, Matsprediktor1/2

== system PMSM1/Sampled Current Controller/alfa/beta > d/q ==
  vect : Inport  Port=1  LatchInput=off
  angle : Inport  Port=2  LatchInput=off
  Fcn : Fcn  Expr=u[1]*cos(u[3])-u[2]*sin(u[3])
  Fcn1 : Fcn  Expr=u[1]*sin(u[3])+u[2]*cos(u[3])
  Mux : Mux  Inputs=2
  Mux1 : Mux  Inputs=2
  Out : Outport  InitialOutput=0
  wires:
  vect/1 -> Mux/1
  angle/1 -> Mux/2
  Mux/1 -> Fcn/1, Fcn1/1
  Fcn/1 -> Mux1/1
  Fcn1/1 -> Mux1/2
  Mux1/1 -> Out/1

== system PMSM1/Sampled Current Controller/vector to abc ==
  vect : Inport  Port=1  LatchInput=off
  Ü> a : Fcn  Expr=sqrt(2/3)*u[1]
  Ü> b : Fcn  Expr=-sqrt(1/6)*u[1]+sqrt(1/2)*u[2]
  Ü> c : Fcn  Expr=-sqrt(1/6)*u[1]-sqrt(1/2)*u[2]
  a : Outport  InitialOutput=0
  b : Outport  Port=2  InitialOutput=0
  c : Outport  Port=3  InitialOutput=0
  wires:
  vect/1 -> Ü> b/1, Ü> a/1, Ü> c/1
  Ü> b/1 -> b/1
  Ü> c/1 -> c/1
  Ü> a/1 -> a/1

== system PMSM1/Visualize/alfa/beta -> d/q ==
  vect : Inport  Port=1  LatchInput=off
  angle : Inport  Port=2  LatchInput=off
  Fcn : Fcn  Expr=u[1]*cos(u[3])-u[2]*sin(u[3])
  Fcn1 : Fcn  Expr=u[1]*sin(u[3])+u[2]*cos(u[3])
  Mux : Mux  Inputs=2
  Mux1 : Mux  Inputs=2
  Out : Outport  InitialOutput=0
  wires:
  vect/1 -> Mux/1
  angle/1 -> Mux/2
  Mux/1 -> Fcn/1, Fcn1/1
  Fcn/1 -> Mux1/1
  Fcn1/1 -> Mux1/2
  Mux1/1 -> Out/1

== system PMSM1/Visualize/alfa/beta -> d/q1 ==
  vect : Inport  Port=1  LatchInput=off
  angle : Inport  Port=2  LatchInput=off
  Fcn : Fcn  Expr=u[1]*cos(u[3])-u[2]*sin(u[3])
  Fcn1 : Fcn  Expr=u[1]*sin(u[3])+u[2]*cos(u[3])
  Mux : Mux  Inputs=2
  Mux1 : Mux  Inputs=2
  Out : Outport  InitialOutput=0
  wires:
  Mux1/1 -> Out/1
  Fcn1/1 -> Mux1/2
  Fcn/1 -> Mux1/1
  Mux/1 -> Fcn1/1, Fcn/1
  angle/1 -> Mux/2
  vect/1 -> Mux/1

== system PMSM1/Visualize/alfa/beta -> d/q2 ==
  vect : Inport  Port=1  LatchInput=off
  angle : Inport  Port=2  LatchInput=off
  Fcn : Fcn  Expr=u[1]*cos(u[3])-u[2]*sin(u[3])
  Fcn1 : Fcn  Expr=u[1]*sin(u[3])+u[2]*cos(u[3])
  Mux : Mux  Inputs=2
  Mux1 : Mux  Inputs=2
  Out : Outport  InitialOutput=0
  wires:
  vect/1 -> Mux/1
  angle/1 -> Mux/2
  Mux/1 -> Fcn/1, Fcn1/1
  Fcn/1 -> Mux1/1
  Fcn1/1 -> Mux1/2
  Mux1/1 -> Out/1

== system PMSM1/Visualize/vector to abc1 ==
  vect : Inport  Port=1  LatchInput=off
  Ü> a : Fcn  Expr=sqrt(2/3)*u[1]
  Ü> b : Fcn  Expr=-sqrt(1/6)*u[1]+sqrt(1/2)*u[2]
  Ü> c : Fcn  Expr=-sqrt(1/6)*u[1]-sqrt(1/2)*u[2]
  a : Outport  InitialOutput=0
  b : Outport  Port=2  InitialOutput=0
  c : Outport  Port=3  InitialOutput=0
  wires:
  Ü> a/1 -> a/1
  Ü> c/1 -> c/1
  Ü> b/1 -> b/1
  vect/1 -> Ü> c/1, Ü> a/1, Ü> b/1

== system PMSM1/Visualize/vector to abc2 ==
  vect : Inport  Port=1  LatchInput=off
  Ü> a : Fcn  Expr=sqrt(2/3)*u[1]
  Ü> b : Fcn  Expr=-sqrt(1/6)*u[1]+sqrt(1/2)*u[2]
  Ü> c : Fcn  Expr=-sqrt(1/6)*u[1]-sqrt(1/2)*u[2]
  a : Outport  InitialOutput=0
  b : Outport  Port=2  InitialOutput=0
  c : Outport  Port=3  InitialOutput=0
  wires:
  vect/1 -> Ü> b/1, Ü> a/1, Ü> c/1
  Ü> b/1 -> b/1
  Ü> c/1 -> c/1
  Ü> a/1 -> a/1

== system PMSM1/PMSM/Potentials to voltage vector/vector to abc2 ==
  vect : Inport  Port=1  LatchInput=off
  Ü> a : Fcn  Expr=sqrt(2/3)*u[1]
  Ü> b : Fcn  Expr=-sqrt(1/6)*u[1]+sqrt(1/2)*u[2]
  Ü> c : Fcn  Expr=-sqrt(1/6)*u[1]-sqrt(1/2)*u[2]
  a : Outport  InitialOutput=0
  b : Outport  Port=2  InitialOutput=0
  c : Outport  Port=3  InitialOutput=0
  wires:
  vect/1 -> Ü> b/1, Ü> a/1, Ü> c/1
  Ü> b/1 -> b/1
  Ü> c/1 -> c/1
  Ü> a/1 -> a/1
